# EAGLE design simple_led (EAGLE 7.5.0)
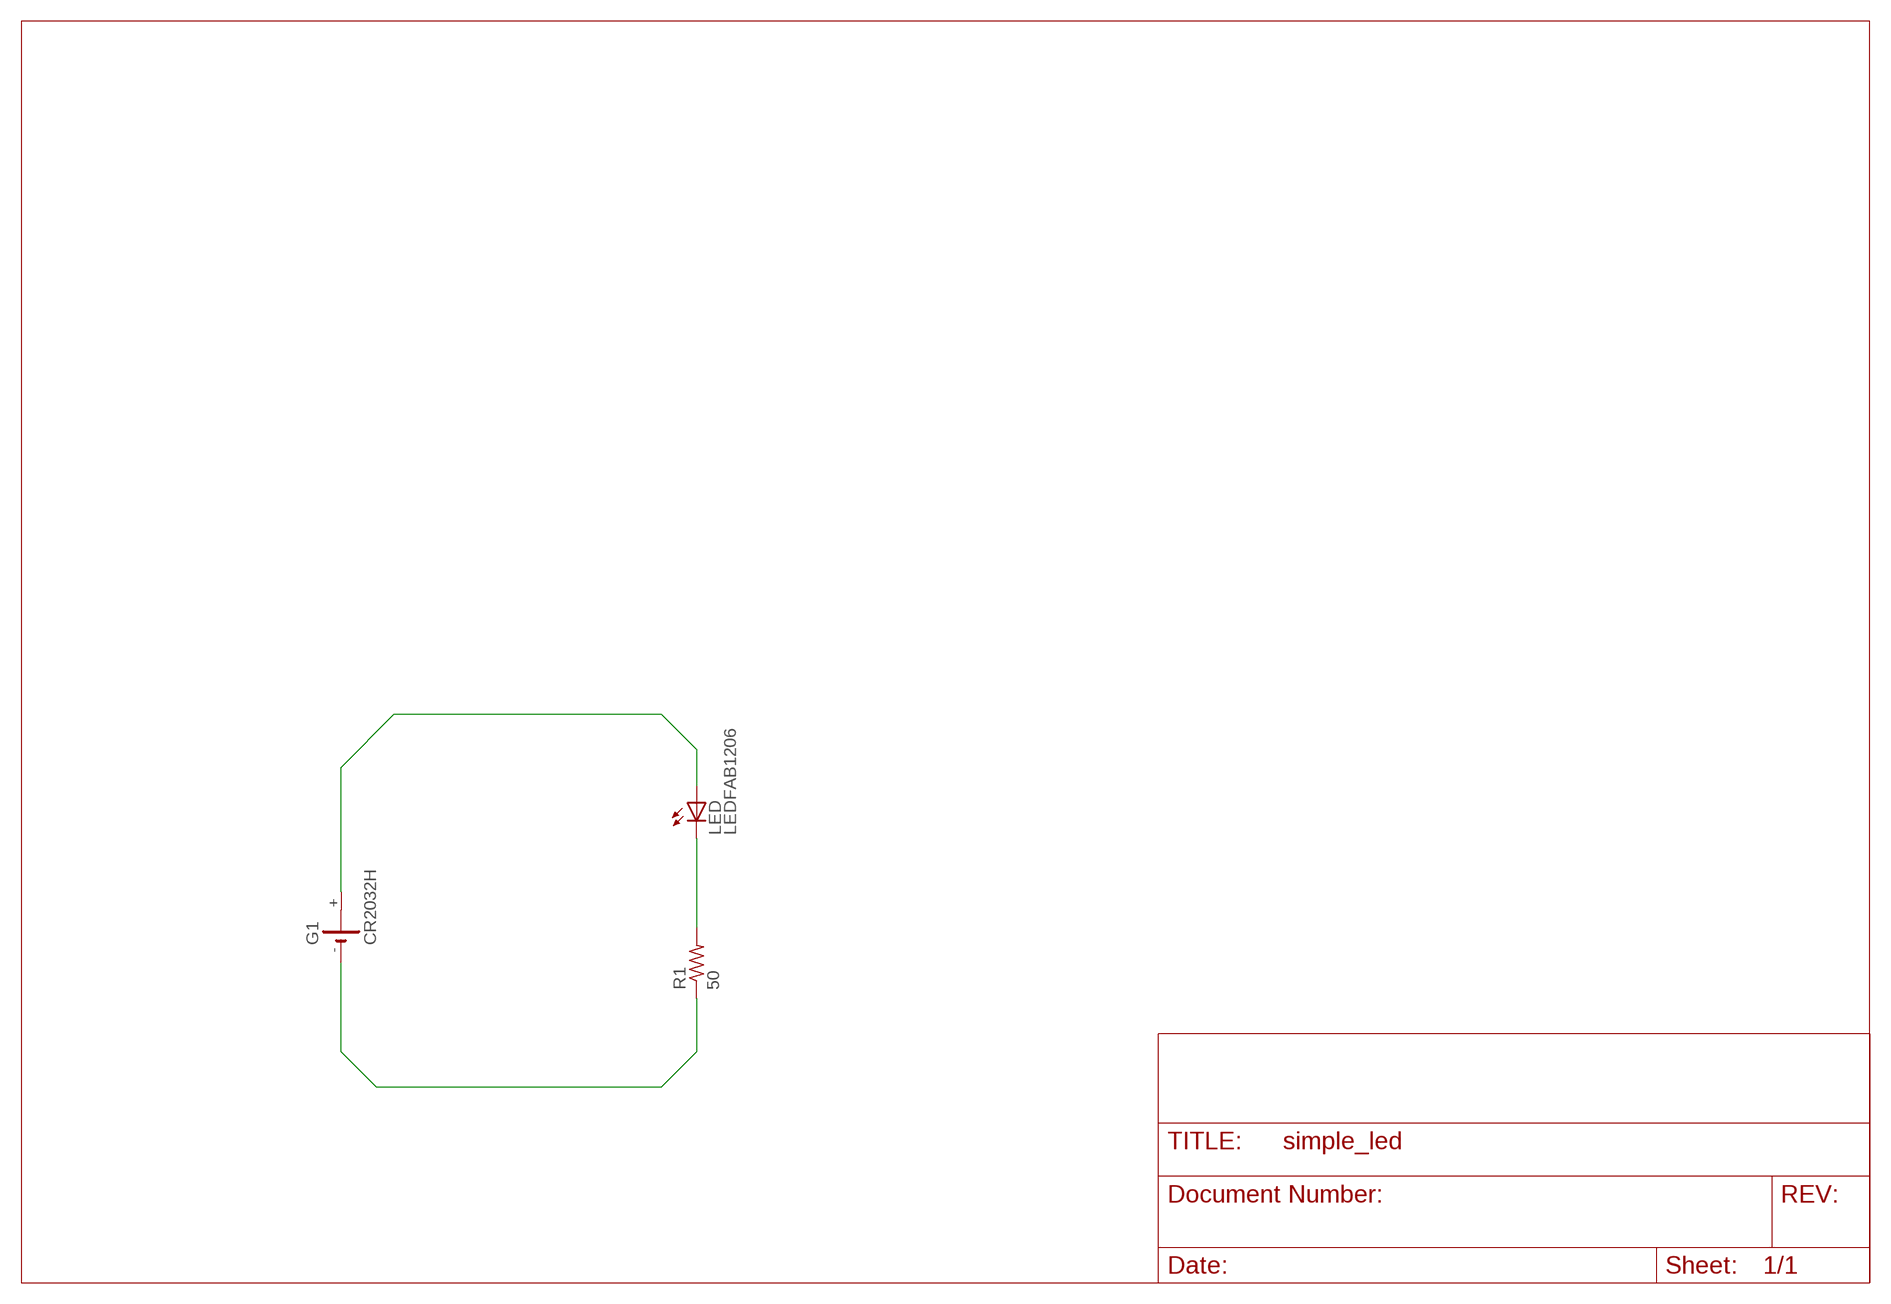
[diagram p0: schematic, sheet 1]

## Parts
G1  CR2032H  [CR2032H]
LED  LEDFAB1206  [LED1206FAB]
R1  50  RES-US1206FAB  [R1206FAB]

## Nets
GND: G1.- R1.1
N$1: G1.+ LED.1(A)
N$2: LED.2(C) R1.2
Unconnected: G1.+@1(+)

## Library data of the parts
G1 = battery:CR2032H: LI BATTERY Varta
LED = fab:LED: LED
R1 = fab:RES-US: Resistor (US Symbol)

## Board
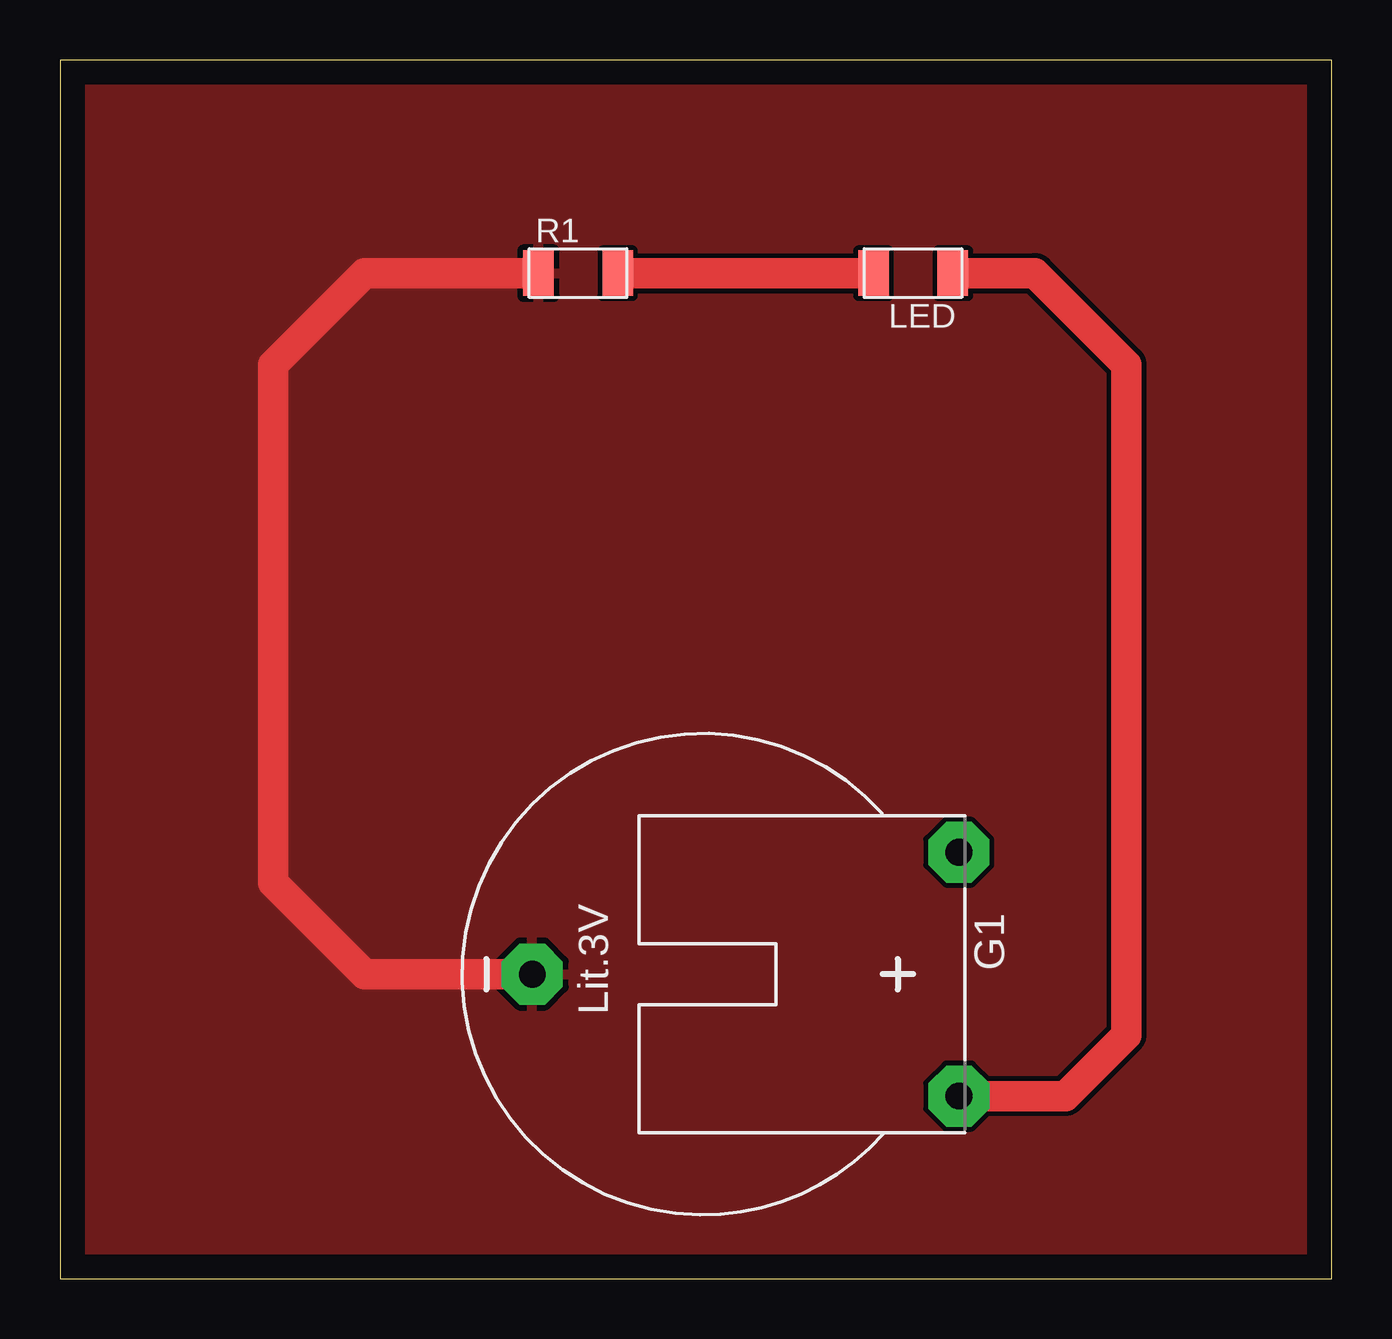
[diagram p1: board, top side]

Size 53.01 x 50.79 mm. Coordinates in mm from the lower left corner, seen from the top.
Outline: 0,0 53.01,0 53.01,50.79 0,50.79 0,0
Copper layers (1*16): Top 0.035mm / dielectric 1.5mm / Bottom 0.035mm
Design rules "default": minimum track width 10mil, minimum drill 24mil, track to track 8mil, track to pad 8mil, pad to pad 8mil, via to via 8mil, smd to smd 8mil, copper to edge 40mil, drill to drill 8mil, minimum pad ring 10mil, minimum via ring 8mil, stop-mask expansion 4mil, vias tented up to drill 0mil, thermal gap 10mil

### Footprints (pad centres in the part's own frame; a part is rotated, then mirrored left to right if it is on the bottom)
CR2032H = drill 1.118 pad 2.54 octagon: + 5.08,10.795; +@1 -5.08,10.795; - 0,-6.985
LED1206FAB = smd 1.27 x 1.905: 1 -1.651,0; 2 1.651,0
R1206FAB = smd 1.27 x 1.905: 1 -1.651,0; 2 1.651,0

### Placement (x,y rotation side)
G1  26.67,12.7 270 top
LED  35.56,41.91 180 top
R1  21.59,41.91 0 top

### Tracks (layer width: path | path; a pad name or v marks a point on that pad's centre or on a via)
GND
  Top 1.27: G1.- 12.7,12.7 8.89,16.51 8.89,38.1 12.7,41.91 R1.1
  pour Top: -6.35,54.61 57.15,54.61 57.15,53.34 57.15,-3.81 -6.35,-3.81
N$1
  Top 1.27: LED.1 40.64,41.91 44.45,38.1 44.45,10.16 41.91,7.62 G1.+
N$2
  Top 1.27: R1.2 LED.2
